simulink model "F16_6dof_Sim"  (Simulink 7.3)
settings: Solver=ode45  StartTime=0.0  StopTime=615.35  RelTol=1e-3
InitFcn:
  | init
StopFcn:
  | pl
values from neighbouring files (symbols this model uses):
  d2r = pi/180    (= 0.0174532925199)    [init.m]    (also in pl.m; LQR_Design.m)
  h0 = 0    [init.m]
  mass = 637    [init.m]
  q = 3    [FCS.m]
  sp = 30    [init.m]
  x0 = 0    [init.m]
  x_cg = -17.29    [init.m]
  x_ref = -17.29    [init.m]
  y_cg = 0    [init.m]
  z_cg = 1.2    [init.m]
undefined symbols (not defined in the file or in its folder): Cl, Cld1, Cld3, Cld4, Cm, Cmd1, Cmd3, Cmd4, Cn, Cnd1, Cnd3, Cnd4, Continuous, CX, CXd1, CXd3, CXd4, CY, CYd1, CYd3, CYd4, CZ, CZd1, CZd3, CZd4, Dryden, F, FCS, ft, km, Light, MIL, r, sigbuilder_block, Thrust
libraries: aerolibasang x3, aerolibwind2 x3, aerolib6dof2 x1, aerolibconvert2 x1, aerolibatmos2 x1, aerolibgravity2 x1, aerolibadyn x1

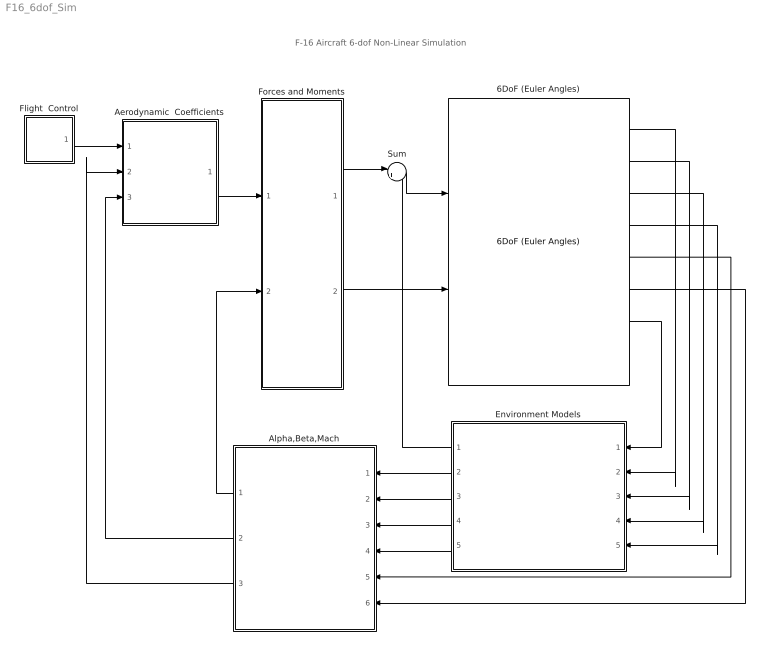
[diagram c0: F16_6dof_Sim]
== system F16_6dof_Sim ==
  note: F-16 Aircraft 6-dof Non-Linear Simulation
  6DoF (Euler Angles) : aerolib6dof2/6DoF (Euler Angles)  SystemSampleTime=-1  units=English (Velocity in ft/s)  mtype=Fixed  rep=Euler Angles  xme_0=[-x0, 0, -h0]  Vm_0=Uvw_0  eul_0=Euler_0  pm_0=pqr_0  mass_0=mass  mass_e=0.5  mass_f=2.0  inertia=inertia  inertia_e=eye(3)  inertia_f=2*eye(3)  k_quat=1.0
  Aerodynamic  Coefficients : Subsystem
  Alpha,Beta,Mach : Subsystem
  Environment Models : Subsystem
  Flight  Control : Subsystem
  Forces and Moments : Subsystem
  Sum : Sum  Inputs=|++  OutDataType=sfix(16)  OutScaling=2^0
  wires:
  6DoF (Euler Angles)/5 -> Alpha,Beta,Mach/5(Vb)
  6DoF (Euler Angles)/1 -> Environment Models/2(Ve)
  6DoF (Euler Angles)/2 -> Environment Models/3(Xe)
  6DoF (Euler Angles)/3 -> Environment Models/4(Euler)
  6DoF (Euler Angles)/4 -> Environment Models/5(DCM)
  Sum/1 -> 6DoF (Euler Angles)/1
  Forces and Moments/1(X,Y,Z) -> Sum/1
  Environment Models/2(Speed of Sound) -> Alpha,Beta,Mach/1(Speed of Sound)
  Environment Models/3(Wind Velocity) -> Alpha,Beta,Mach/2(Wind Velocity)
  Environment Models/4(Air Density) -> Alpha,Beta,Mach/3(Air Density)
  Environment Models/5(Wind Angular Rates) -> Alpha,Beta,Mach/4(Wind Angular Rates)
  Environment Models/1(Fg) -> Sum/2
  Alpha,Beta,Mach/1(qbar) -> Forces and Moments/2(qbar)
  Alpha,Beta,Mach/3(Incid) -> Aerodynamic  Coefficients/2(Incid)
  Alpha,Beta,Mach/2(Mach) -> Aerodynamic  Coefficients/3(Mach)
  6DoF (Euler Angles)/6 -> Alpha,Beta,Mach/6(p,q,r)
  Aerodynamic  Coefficients/1(Coeff) -> Forces and Moments/1(Coeff)
  Forces and Moments/2(LMN) -> 6DoF (Euler Angles)/2
  Flight  Control/1(Deltas) -> Aerodynamic  Coefficients/1(deltas)
  6DoF (Euler Angles)/7 -> Environment Models/1(omgd)

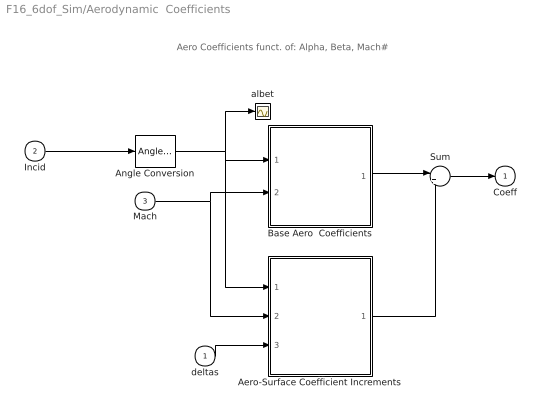
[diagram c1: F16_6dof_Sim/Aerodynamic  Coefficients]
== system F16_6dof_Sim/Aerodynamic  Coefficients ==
  note: Aero Coefficients funct. of: Alpha, Beta, Mach#
  deltas : Inport  OutDataType=sfix(16)  OutScaling=2^0
  Incid : Inport  Port=2  OutDataType=sfix(16)  OutScaling=2^0
  Mach : Inport  Port=3  OutDataType=sfix(16)  OutScaling=2^0
  Aero-Surface Coefficient Increments : Subsystem
  Angle Conversion : aerolibconvert2/Angle Conversion  SystemSampleTime=-1  IU=rad  OU=deg
  Base Aero  Coefficients : Subsystem
  Sum : Sum  Inputs=|++  OutDataType=fixdt(1, 16)  OutScaling=2^0
  albet : Scope
  Coeff : Outport  OutDataType=sfix(16)  OutScaling=2^0  InitialOutput=0
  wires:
  Incid/1 -> Angle Conversion/1
  Angle Conversion/1 -> albet/1, Base Aero  Coefficients/1(albet), Aero-Surface Coefficient Increments/1(albet)
  Mach/1 -> Base Aero  Coefficients/2(Mach), Aero-Surface Coefficient Increments/2(Mach)
  Sum/1 -> Coeff/1
  Base Aero  Coefficients/1(Coeff) -> Sum/1
  Aero-Surface Coefficient Increments/1(Coeff) -> Sum/2
  deltas/1 -> Aero-Surface Coefficient Increments/3(delta)

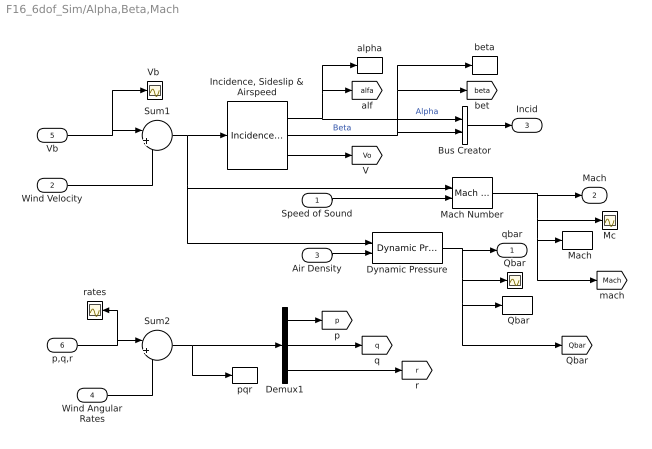
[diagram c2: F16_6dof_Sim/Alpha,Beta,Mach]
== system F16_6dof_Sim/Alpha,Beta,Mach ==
  Speed of Sound : Inport  OutDataType=sfix(16)  OutScaling=2^0
  Wind Velocity : Inport  Port=2  PortDimensions=3  OutDataType=sfix(16)  OutScaling=2^0
  Air Density : Inport  Port=3  OutDataType=sfix(16)  OutScaling=2^0
  Wind Angular Rates : Inport  Port=4  PortDimensions=3  OutDataType=sfix(16)  OutScaling=2^0
  Vb : Inport  Port=5  PortDimensions=3  OutDataType=sfix(16)  OutScaling=2^0
  p,q,r : Inport  Port=6  PortDimensions=3  OutDataType=sfix(16)  OutScaling=2^0
  "  Mach" : ToWorkspace  VariableName=Mach  SampleTime=-1  SaveFormat=Array
  " Qbar" : ToWorkspace  VariableName=Qbar  SampleTime=-1  SaveFormat=Array
  Bus Creator : BusCreator  Inputs=2
  Demux1 : Demux  Outputs=3
  Dynamic Pressure : aerolibasang/Dynamic Pressure  SystemSampleTime=-1
  "Incidence, Sideslip & Airspeed" : aerolibasang/Incidence, Sideslip, & Airspeed  SystemSampleTime=-1
  Mach Number : aerolibasang/Mach Number  SystemSampleTime=-1
  Mc : Scope
  Qbar : Scope
  Sum1 : Sum  Inputs=|+-  OutDataType=sfix(16)  OutScaling=2^0
  Sum2 : Sum  Inputs=|++  OutDataType=sfix(16)  OutScaling=2^0
  "Vb " : Scope
  alpha : ToWorkspace  VariableName=alfa  SampleTime=-1  SaveFormat=Array
  beta : ToWorkspace  VariableName=beta  SampleTime=-1  SaveFormat=Array
  pqr : ToWorkspace  VariableName=pqr  SampleTime=-1  SaveFormat=Array
  rates : Scope
  qbar : Outport  OutDataType=sfix(16)  OutScaling=2^0  InitialOutput=0
  Mach : Outport  Port=2  OutDataType=sfix(16)  OutScaling=2^0
  Incid : Outport  Port=3  OutDataType=sfix(16)  OutScaling=2^0
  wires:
  "Incidence, Sideslip & Airspeed"/3 -> [Vo]
  Dynamic Pressure/1 -> qbar/1, Qbar/1, " Qbar"/1, [Qbar]
  Air Density/1 -> Dynamic Pressure/2
  Mach Number/1 -> Mach/1, Mc/1, "  Mach"/1, [Mach]
  Sum1/1 -> Dynamic Pressure/1, Mach Number/1, "Incidence, Sideslip & Airspeed"/1
  Vb/1 -> Sum1/1, "Vb "/1
  Speed of Sound/1 -> Mach Number/2
  Wind Velocity/1 -> Sum1/2
  "Incidence, Sideslip & Airspeed"/2 -> Bus Creator/2, [beta], beta/1  "Beta"
  Bus Creator/1 -> Incid/1
  "Incidence, Sideslip & Airspeed"/1 -> Bus Creator/1, [alfa], alpha/1  "Alpha"
  p,q,r/1 -> Sum2/1, rates/1
  Wind Angular Rates/1 -> Sum2/2
  Sum2/1 -> Demux1/1, pqr/1
  Demux1/2 -> [q]
  Demux1/3 -> [r]
  Demux1/1 -> [p]

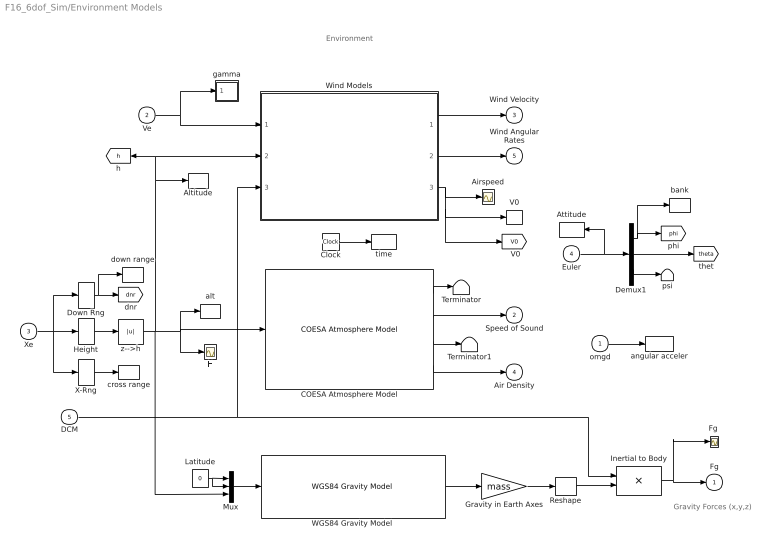
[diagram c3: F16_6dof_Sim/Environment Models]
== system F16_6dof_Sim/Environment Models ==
  note: Gravity Forces (x,y,z)
  note: Environment
  omgd : Inport  OutDataType=sfix(16)  OutScaling=2^0
  Ve : Inport  Port=2  OutDataType=sfix(16)  OutScaling=2^0
  Xe : Inport  Port=3  PortDimensions=3  OutDataType=sfix(16)  OutScaling=2^0
  Euler : Inport  Port=4  OutDataType=sfix(16)  OutScaling=2^0
  DCM : Inport  Port=5  OutDataType=sfix(16)  OutScaling=2^0
  Airspeed : Scope
  Altitude : ToWorkspace  VariableName=Alt  SampleTime=-1  SaveFormat=Array
  Attitude : ToWorkspace  VariableName=Euler  SampleTime=-1  SaveFormat=Array
  COESA Atmosphere Model : aerolibatmos2/COESA Atmosphere Model  SystemSampleTime=-1  units=English (Velocity in ft/s)  spec=1976 COESA-extended U.S. Standard Atmosphere  model=Profile  profile_var=High temperature  profile_percent=1%  profile_alt=5 km (16404 ft)  envelope_var=High temperature  envelope_percent=1%  action=Warning
  Clock : Clock
  Demux1 : Demux  Outputs=3
  Down Rng : Selector  InputPortWidth=3  IndexOptions=Index vector (dialog)  Indices=[1]  OutputSizes=1
  "Fg " : Scope
  Gravity in Earth Axes : Gain  Gain=mass  ParameterDataType=sfix(16)  ParameterScaling=2^0  OutDataType=sfix(16)  OutScaling=2^0
  H : Scope
  Height : Selector  InputPortWidth=3  IndexOptions=Index vector (dialog)  Indices=[3]  OutputSizes=1
  Inertial to Body : Product  Multiplication=Matrix(*)  OutDataType=sfix(16)  OutScaling=2^0
  Latitude : Constant  Value=0  OutDataType=sfix(16)  OutScaling=2^0
  Mux : Mux  Inputs=3
  Reshape : Reshape
  Terminator : Terminator
  Terminator1 : Terminator
  V0 : ToWorkspace  VariableName=V0  SampleTime=-1  SaveFormat=Array
  "WGS84 Gravity Model " : aerolibgravity2/WGS84 Gravity Model   SystemSampleTime=-1  model=WGS84 Taylor Series  units=English  no_atmos=on  precessing=on  jd_loc=off  month=October  day=10  year=2004  no_centrifugal=on  action=None
  Wind Models : Subsystem
  X-Rng : Selector  InputPortWidth=3  IndexOptions=Index vector (dialog)  Indices=[2]  OutputSizes=1
  alt : ToWorkspace  VariableName=alt  SampleTime=-1  SaveFormat=Array
  angular acceler : ToWorkspace  VariableName=omgd  SampleTime=-1  SaveFormat=Array
  bank : ToWorkspace  VariableName=phi  SampleTime=-1  SaveFormat=Array
  cross range : ToWorkspace  VariableName=xrng  SampleTime=-1  SaveFormat=Array
  down range : ToWorkspace  VariableName=dnr  SampleTime=-1  SaveFormat=Array
  gamma : Subsystem
  psi : Terminator
  time : ToWorkspace  VariableName=time  SampleTime=-1  SaveFormat=Array
  z-->h : Abs
  Fg : Outport  OutDataType=sfix(16)  OutScaling=2^0  InitialOutput=0
  Speed of Sound : Outport  Port=2  OutDataType=sfix(16)  OutScaling=2^0  InitialOutput=0
  Wind Velocity : Outport  Port=3  OutDataType=sfix(16)  OutScaling=2^0  InitialOutput=0
  Air Density : Outport  Port=4  OutDataType=sfix(16)  OutScaling=2^0  InitialOutput=0
  Wind Angular Rates : Outport  Port=5  OutDataType=sfix(16)  OutScaling=2^0  InitialOutput=0
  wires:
  Reshape/1 -> Inertial to Body/2
  "WGS84 Gravity Model "/1 -> Gravity in Earth Axes/1
  Gravity in Earth Axes/1 -> Reshape/1
  COESA Atmosphere Model/1 -> Terminator/1
  COESA Atmosphere Model/2 -> Speed of Sound/1
  COESA Atmosphere Model/3 -> Terminator1/1
  COESA Atmosphere Model/4 -> Air Density/1
  DCM/1 -> Inertial to Body/1, Wind Models/3(DCM)
  Inertial to Body/1 -> Fg/1, "Fg "/1
  Mux/1 -> "WGS84 Gravity Model "/1
  Latitude/1 -> Mux/2, Mux/1
  Height/1 -> z-->h/1
  Xe/1 -> Height/1, Down Rng/1, X-Rng/1
  z-->h/1 -> COESA Atmosphere Model/1, H/1, alt/1, Mux/3, Wind Models/2(Altitude), [h], Altitude/1
  Wind Models/2(pg,qg,rg) -> Wind Angular Rates/1
  Wind Models/3(Airspeed) -> Airspeed/1, V0/1, [V0]
  Ve/1 -> Wind Models/1(Ve), gamma/1(Ve)
  Wind Models/1(ug,vg,wg) -> Wind Velocity/1
  Down Rng/1 -> [dnr], down range/1
  Clock/1 -> time/1
  X-Rng/1 -> cross range/1
  omgd/1 -> angular acceler/1
  Euler/1 -> Demux1/1, Attitude/1
  Demux1/2 -> [theta]
  Demux1/1 -> [phi], bank/1
  Demux1/3 -> psi/1

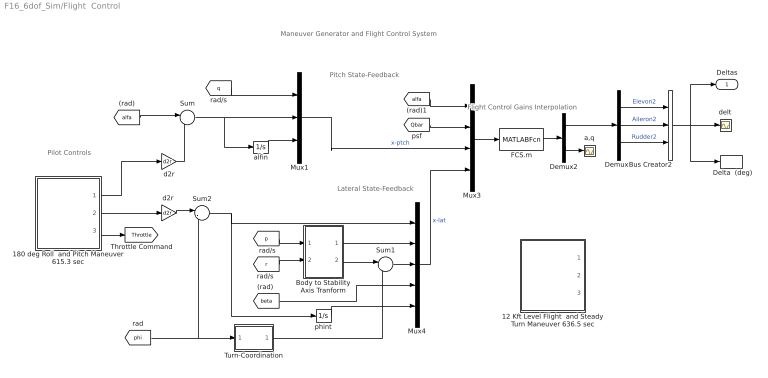
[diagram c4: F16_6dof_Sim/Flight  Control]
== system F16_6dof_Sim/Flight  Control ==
  note: Maneuver Generator and Flight Control System
  note: Flight Control Gains Interpolation
  note: Pilot Controls
  note: Pitch State-Feedback
  note: Lateral State-Feedback
  "  Delta  (deg)" : ToWorkspace  VariableName=delta  SampleTime=-1  SaveFormat=Array
  12 Kft Level Flight  and Steady Turn Maneuver 636.5 sec : Subsystem  Tag=STV Subsys  LoadFcn=sigbuilder_block('load');  StartFcn=sigbuilder_block('start');  StopFcn=sigbuilder_block('stop');  ClipboardFcn=sigbuilder_block('clipboard');
  180 deg Roll  and Pitch Maneuver 615.3 sec : Subsystem  Tag=STV Subsys  LoadFcn=sigbuilder_block('load');  StartFcn=sigbuilder_block('start');  StopFcn=sigbuilder_block('stop');  ClipboardFcn=sigbuilder_block('clipboard');
  Body to Stability Axis Tranform : Subsystem
  Bus Creator2 : BusCreator  Inputs=3
  Demux1 : Demux  Outputs=3
  Demux2 : Demux  Outputs=[3,2]
  FCS.m : MATLABFcn  MATLABFcn=FCS( u(1), u(2), u(3:5), u(6:10) )  OutputDimensions=5
  Mux1 : Mux  Inputs=3
  Mux3 : Mux  Inputs=[1,1, 3, 5]
  Mux4 : Mux  Inputs=5
  Sum : Sum  Inputs=|+-  OutDataType=fixdt(1, 16)  OutScaling=2^0
  Sum1 : Sum  Inputs=|++  OutDataType=fixdt(1, 16)  OutScaling=2^0
  Sum2 : Sum  Inputs=|-+  OutDataType=fixdt(1, 16)  OutScaling=2^0
  Turn-Coordination : Subsystem
  a,q : Scope
  alfin : Integrator
  d2r : Gain  Gain=d2r  ParameterDataType=fixdt(1, 16)  ParameterScaling=2^0  OutDataType=fixdt(1, 16)  OutScaling=2^0
  "d2r " : Gain  Gain=d2r  ParameterDataType=fixdt(1, 16)  ParameterScaling=2^0  OutDataType=fixdt(1, 16)  OutScaling=2^0
  delt : Scope
  phint : Integrator
  Deltas : Outport
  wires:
  Mux1/1 -> Mux3/3  "x-ptch"
  [q] -> Mux1/1
  alfin/1 -> Mux1/3
  Sum/1 -> Mux1/2, alfin/1
  [alfa] -> Sum/1
  d2r/1 -> Sum/2
  Sum2/1 -> phint/1, Mux4/1
  [beta] -> Mux4/4
  phint/1 -> Mux4/5
  180 deg Roll  and Pitch Maneuver 615.3 sec/2(Phi_cmd) -> "d2r "/1
  180 deg Roll  and Pitch Maneuver 615.3 sec/1(Alpha_cmd) -> d2r/1
  180 deg Roll  and Pitch Maneuver 615.3 sec/3(Throttle) -> [Throttle]
  Demux1/1 -> Bus Creator2/1  "Elevon2"
  Bus Creator2/1 -> delt/1, Deltas/1, "  Delta  (deg)"/1
  Demux1/2 -> Bus Creator2/2  "Aileron2"
  Demux1/3 -> Bus Creator2/3  "Rudder2"
  FCS.m/1 -> Demux2/1
  Demux2/1 -> Demux1/1
  Demux2/2 -> a,q/1
  [alfa] -> Mux3/1
  [Qbar] -> Mux3/2
  "d2r "/1 -> Sum2/1
  [phi] -> Sum2/2, Turn-Coordination/1(phi)
  Sum1/1 -> Mux4/3
  Turn-Coordination/1(Rff) -> Sum1/2
  Body to Stability Axis Tranform/2(r_s) -> Sum1/1
  Body to Stability Axis Tranform/1(p_s) -> Mux4/2
  [p] -> Body to Stability Axis Tranform/1(p_b)
  [r] -> Body to Stability Axis Tranform/2(r_b)
  Mux4/1 -> Mux3/4  "x-lat"
  Mux3/1 -> FCS.m/1

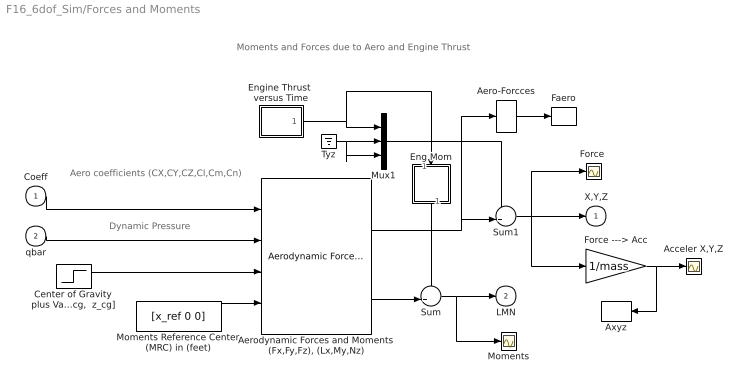
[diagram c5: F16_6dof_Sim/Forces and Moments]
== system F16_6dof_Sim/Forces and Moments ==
  note: Aero coefficients (CX,CY,CZ,Cl,Cm,Cn)
  note: Dynamic Pressure
  note: Moments and Forces due to Aero and Engine Thrust
  Coeff : Inport  OutDataType=sfix(16)  OutScaling=2^0
  qbar : Inport  Port=2  OutDataType=sfix(16)  OutScaling=2^0
  Acceler X,Y,Z : Scope
  Aero-Forcces : Selector  InputPortWidth=3  IndexOptions=Index vector (dialog)  Indices=[3,1,2]  OutputSizes=1
  "Aerodynamic Forces and Moments (Fx,Fy,Fz), (Lx,My,Nz)" : aerolibadyn/Aerodynamic Forces and Moments   SystemSampleTime=-1  inputAxes=Body  outputForceAxes=Body  outputMomentAxes=Body  S=Sref  b=sp  cbar=ch
  Axyz : ToWorkspace  VariableName=Axyz  SampleTime=-1  SaveFormat=Array
  "Center of Gravity plus Variation [x_cg, y_cg,  z_cg]" : Step  Time=100*[1 1 1]  Before="[x_cg, y_cg,  z_cg]"  After="[x_cg,   y_cg+0.0,   z_cg]"
  Eng Mom : Subsystem
  Engine Thrust  versus Time : Subsystem
  Faero : ToWorkspace  VariableName=Flds  SampleTime=-1  SaveFormat=Array
  "Force " : Scope
  Force ---> Acc : Gain  Gain=1/mass  ParameterDataType=sfix(16)  ParameterScaling=2^0  OutDataType=sfix(16)  OutScaling=2^0
  Moments : Scope
  Moments Reference Center (MRC) in (feet) : Constant  Value=[x_ref 0 0]  OutDataType=sfix(16)  OutScaling=2^0
  Mux1 : Mux  Inputs=3
  Sum : Sum  Inputs=++|  OutDataType=fixdt(1, 16)  OutScaling=2^0
  Sum1 : Sum  Inputs=++|  OutDataType=sfix(16)  OutScaling=2^0
  Tyz : Ground
  X,Y,Z : Outport  OutDataType=sfix(16)  OutScaling=2^0  InitialOutput=0
  LMN : Outport  Port=2  OutDataType=sfix(16)  OutScaling=2^0  InitialOutput=0
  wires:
  Coeff/1 -> "Aerodynamic Forces and Moments (Fx,Fy,Fz), (Lx,My,Nz)"/1
  qbar/1 -> "Aerodynamic Forces and Moments (Fx,Fy,Fz), (Lx,My,Nz)"/2
  Sum1/1 -> Force ---> Acc/1, X,Y,Z/1, "Force "/1
  Moments Reference Center (MRC) in (feet)/1 -> "Aerodynamic Forces and Moments (Fx,Fy,Fz), (Lx,My,Nz)"/4
  "Center of Gravity plus Variation [x_cg, y_cg,  z_cg]"/1 -> "Aerodynamic Forces and Moments (Fx,Fy,Fz), (Lx,My,Nz)"/3
  Force ---> Acc/1 -> Acceler X,Y,Z/1, Axyz/1
  Mux1/1 -> Sum1/1
  Tyz/1 -> Mux1/2, Mux1/3
  Engine Thrust  versus Time/1(Thrust) -> Mux1/1, Eng Mom/1(Te)
  Aero-Forcces/1 -> Faero/1
  "Aerodynamic Forces and Moments (Fx,Fy,Fz), (Lx,My,Nz)"/2 -> Sum/2
  "Aerodynamic Forces and Moments (Fx,Fy,Fz), (Lx,My,Nz)"/1 -> Sum1/2, Aero-Forcces/1
  Eng Mom/1(Me) -> Sum/1
  Sum/1 -> LMN/1, Moments/1

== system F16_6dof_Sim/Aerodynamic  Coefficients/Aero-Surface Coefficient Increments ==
  note: Surface Coefficients
  albet : Inport
  Mach : Inport  Port=2
  delta : Inport  Port=3
  Aileron : Subsystem
  Elevon : Subsystem
  Rudder : Subsystem
  Sum : Sum  Inputs=+++  OutDataType=fixdt(1, 16)  OutScaling=2^0
  Coeff : Outport
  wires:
  Elevon/1(Coeff) -> Sum/1
  delta/1 -> Elevon/3(delta), Aileron/3(delta), Rudder/3(delta)
  albet/1 -> Elevon/1(albet), Aileron/1(albet), Rudder/1(albet)
  Mach/1 -> Elevon/2(Mach), Aileron/2(Mach), Rudder/2(Mach)
  Sum/1 -> Coeff/1
  Aileron/1(Coeff) -> Sum/2
  Rudder/1(Coeff) -> Sum/3

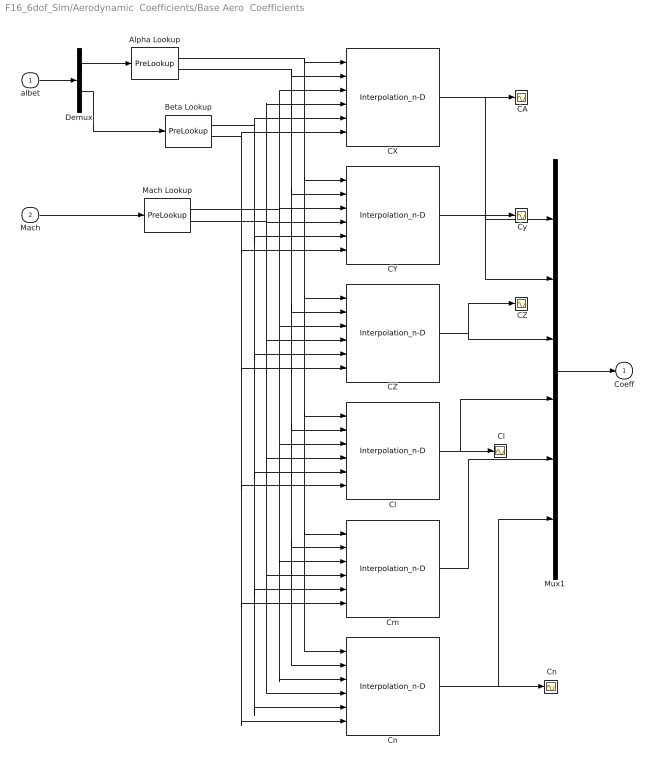
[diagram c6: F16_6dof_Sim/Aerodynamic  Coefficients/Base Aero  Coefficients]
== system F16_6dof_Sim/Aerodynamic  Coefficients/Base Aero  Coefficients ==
  albet : Inport  OutDataType=sfix(16)  OutScaling=2^0
  Mach : Inport  Port=2  OutDataType=sfix(16)  OutScaling=2^0
  " CA" : Scope
  " CZ" : Scope
  " Cl" : Scope
  " Cn" : Scope
  " Cy" : Scope
  Alpha Lookup : PreLookup  BreakpointsData=Alfas  BeginIndexSearchUsingPreviousIndexResult=on  ProcessOutOfRangeInput=Linear extrapolation  IndexDataType=sfix(16)  FractionDataType=sfix(16)  FractionScaling=2^0
  Beta Lookup : PreLookup  BreakpointsData=Betas  BeginIndexSearchUsingPreviousIndexResult=on  ProcessOutOfRangeInput=Linear extrapolation  IndexDataType=sfix(16)  FractionDataType=sfix(16)  FractionScaling=2^0
  CX : Interpolation_n-D  NumberOfTableDimensions=3  Table=CX  CheckIndexInCode=off  OutDataType=sfix(16)  OutScaling=2^0
  CY : Interpolation_n-D  NumberOfTableDimensions=3  Table=CY  CheckIndexInCode=off  OutDataType=sfix(16)  OutScaling=2^0
  CZ : Interpolation_n-D  NumberOfTableDimensions=3  Table=CZ  CheckIndexInCode=off  OutDataType=sfix(16)  OutScaling=2^0
  Cl : Interpolation_n-D  NumberOfTableDimensions=3  Table=Cl  CheckIndexInCode=off  OutDataTypeMode=double  OutDataType=sfix(16)  OutScaling=2^0  OutDataTypeStr=double
  Cm : Interpolation_n-D  NumberOfTableDimensions=3  Table=Cm  CheckIndexInCode=off  OutDataType=sfix(16)  OutScaling=2^0
  Cn : Interpolation_n-D  NumberOfTableDimensions=3  Table=Cn  CheckIndexInCode=off  OutDataType=sfix(16)  OutScaling=2^0
  Demux : Demux  Outputs=2
  Mach Lookup : PreLookup  BreakpointsData=Machs  BeginIndexSearchUsingPreviousIndexResult=on  ProcessOutOfRangeInput=Linear extrapolation  IndexDataType=sfix(16)  FractionDataType=sfix(16)  FractionScaling=2^0
  Mux1 : Mux  Inputs=6
  Coeff : Outport  OutDataType=sfix(16)  OutScaling=2^0  InitialOutput=0
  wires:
  Demux/1 -> Alpha Lookup/1
  CX/1 -> Mux1/1, " CA"/1
  CY/1 -> Mux1/2, " Cy"/1
  CZ/1 -> Mux1/3, " CZ"/1
  Cl/1 -> Mux1/4, " Cl"/1
  Cm/1 -> Mux1/5
  Cn/1 -> Mux1/6, " Cn"/1
  Alpha Lookup/1 -> CX/1, CY/1, Cm/1, Cn/1, Cl/1, CZ/1
  Alpha Lookup/2 -> CX/2, CY/2, CZ/2, Cl/2, Cm/2, Cn/2
  Mach Lookup/1 -> CY/3, Cm/3, Cn/3, Cl/3, CZ/3, CX/3
  Mach Lookup/2 -> CY/4, Cm/4, Cn/4, Cl/4, CZ/4, CX/4
  Beta Lookup/1 -> CX/5, Cm/5, Cn/5, Cl/5, CZ/5, CY/5
  Beta Lookup/2 -> CX/6, CY/6, Cm/6, Cn/6, Cl/6, CZ/6
  Mux1/1 -> Coeff/1
  Demux/2 -> Beta Lookup/1
  albet/1 -> Demux/1
  Mach/1 -> Mach Lookup/1

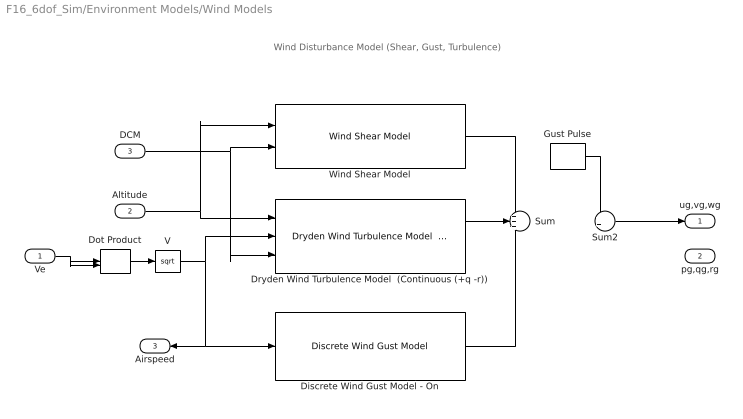
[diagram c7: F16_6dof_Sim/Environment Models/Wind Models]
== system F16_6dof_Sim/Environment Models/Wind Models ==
  note: Wind Disturbance Model (Shear, Gust, Turbulence)
  Ve : Inport  OutDataType=sfix(16)  OutScaling=2^0
  Altitude : Inport  Port=2  OutDataType=sfix(16)  OutScaling=2^0
  DCM : Inport  Port=3  OutDataType=sfix(16)  OutScaling=2^0
  Discrete Wind Gust Model - On : aerolibwind2/Discrete Wind Gust Model  SystemSampleTime=-1  units=English (Velocity in ft/s)  Gx=on  Gy=on  Gz=on  t_0=20  d_m=[120 120 80]  v_m=[3.5 3.0 3.0]
  Dot Product : DotProduct  OutDataType=sfix(16)  OutScaling=2^-10  SaturateOnIntegerOverflow=on
  Dryden Wind Turbulence Model  (Continuous (+q -r)) : aerolibwind2/Dryden Wind Turbulence Model  (Continuous (+q -r))  SystemSampleTime=-1  units=English (Velocity in ft/s)  spec=MIL-F-8785C  model=Continuous Dryden (+q -r)  W20=5  Wdeg=0  TurbProb=10^-2 - Light  L_high=533.4  Wingspan=4  ts=0.1  Seed=[23341 23342 23343 23344]  T_on=on
  Gust Pulse : DiscretePulseGenerator  PulseType=Time based  Amplitude=[0, 0, 0]  Period=[100, 100, 100]  PulseWidth=1  PhaseDelay=0  SampleTime=1
  Sum : Sum  Inputs=+++  OutDataType=sfix(16)  OutScaling=2^0
  Sum2 : Sum  Inputs=++|  OutDataType=sfix(16)  OutScaling=2^0
  V : Math  Operator=sqrt  OutDataType=sfix(16)  OutScaling=2^0
  Wind Shear Model : aerolibwind2/Wind Shear Model  SystemSampleTime=-1  units=English (Velocity in ft/s)  phase=Category C - Terminal Flight Phase  W_20=1  Wdeg=0
  ug,vg,wg : Outport  OutDataType=sfix(16)  OutScaling=2^0
  pg,qg,rg : Outport  Port=2  OutDataType=sfix(16)  OutScaling=2^0
  Airspeed : Outport  Port=3  OutDataType=sfix(16)  OutScaling=2^0
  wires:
  Dryden Wind Turbulence Model  (Continuous (+q -r))/1 -> Sum/2
  Discrete Wind Gust Model - On/1 -> Sum/3
  Wind Shear Model/1 -> Sum/1
  DCM/1 -> Wind Shear Model/2, Dryden Wind Turbulence Model  (Continuous (+q -r))/3
  Altitude/1 -> Dryden Wind Turbulence Model  (Continuous (+q -r))/1, Wind Shear Model/1
  Dot Product/1 -> V/1
  Ve/1 -> Dot Product/1, Dot Product/2
  V/1 -> Dryden Wind Turbulence Model  (Continuous (+q -r))/2, Discrete Wind Gust Model - On/1, Airspeed/1
  Sum2/1 -> ug,vg,wg/1
  Gust Pulse/1 -> Sum2/1
  Sum/1 -> ?
  Dryden Wind Turbulence Model  (Continuous (+q -r))/2 -> ?

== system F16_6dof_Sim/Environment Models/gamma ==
  Ve : Inport
  -1 : Gain  Gain=-1  ParameterDataType=sfix(16)  ParameterScaling=2^0  OutDataType=sfix(16)  OutScaling=2^0
  57.2 : Gain  Gain=180/pi  ParameterDataType=sfix(16)  ParameterScaling=2^0  OutDataType=sfix(16)  OutScaling=2^0
  Vx : Selector  InputPortWidth=3  IndexOptions=Index vector (dialog)  Indices=[1]  OutputSizes=1
  Vz : Selector  InputPortWidth=3  IndexOptions=Index vector (dialog)  Indices=[3]  OutputSizes=1
  atan : Trigonometry  Operator=atan2
  "gam " : Scope
  gama : ToWorkspace  VariableName=gama  SampleTime=-1  SaveFormat=Array
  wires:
  Vz/1 -> atan/1
  Vx/1 -> atan/2
  atan/1 -> 57.2/1
  57.2/1 -> "gam "/1, gama/1
  -1/1 -> Vz/1
  Ve/1 -> -1/1, Vx/1

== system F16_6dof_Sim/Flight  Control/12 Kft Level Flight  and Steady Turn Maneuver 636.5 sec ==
  Demux : Demux  Tag=STV Demux  Outputs=3
  FromWs : FromWorkspace  Tag=STV FromWs  VariableName=tuvar  SampleTime=0  SigBuilderData=DataTag0  VnvData=DataTag1
  Alpha_cmd : Outport  Tag=STV Outport
  Phi_cmd : Outport  Tag=STV Outport  Port=2
  Throttle : Outport  Tag=STV Outport  Port=3
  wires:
  FromWs/1 -> Demux/1
  Demux/1 -> Alpha_cmd/1
  Demux/2 -> Phi_cmd/1
  Demux/3 -> Throttle/1

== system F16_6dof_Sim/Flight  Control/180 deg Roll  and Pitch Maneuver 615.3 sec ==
  Demux : Demux  Tag=STV Demux  Outputs=3
  FromWs : FromWorkspace  Tag=STV FromWs  VariableName=tuvar  SampleTime=0  SigBuilderData=DataTag2  VnvData=DataTag3
  Alpha_cmd : Outport  Tag=STV Outport
  Phi_cmd : Outport  Tag=STV Outport  Port=2
  Throttle : Outport  Tag=STV Outport  Port=3
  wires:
  FromWs/1 -> Demux/1
  Demux/1 -> Alpha_cmd/1
  Demux/2 -> Phi_cmd/1
  Demux/3 -> Throttle/1

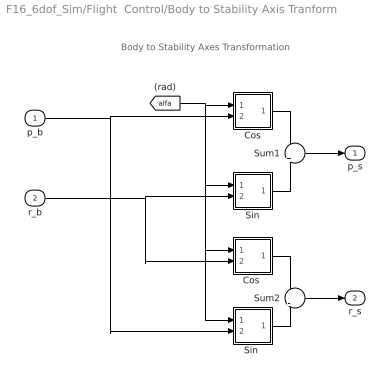
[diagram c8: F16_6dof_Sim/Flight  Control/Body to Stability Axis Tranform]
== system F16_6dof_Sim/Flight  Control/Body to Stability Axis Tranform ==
  note: Body to Stability Axes Transformation
  p_b : Inport  OutDataType=sfix(16)  OutScaling=2^0
  r_b : Inport  Port=2  OutDataType=sfix(16)  OutScaling=2^0
  Cos : Subsystem
  "Cos " : Subsystem
  Sin : Subsystem
  "Sin " : Subsystem
  Sum1 : Sum  Inputs=+|+  OutDataType=sfix(16)  OutScaling=2^0
  Sum2 : Sum  Inputs=+|-  OutDataType=sfix(16)  OutScaling=2^0
  p_s : Outport  OutDataType=sfix(16)  OutScaling=2^0
  r_s : Outport  Port=2  OutDataType=sfix(16)  OutScaling=2^0
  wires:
  Sum1/1 -> p_s/1
  Sum2/1 -> r_s/1
  p_b/1 -> Cos/2(in), "Sin "/2(in)
  r_b/1 -> Sin/2(in), "Cos "/2(in)
  Sin/1(sa) -> Sum1/2
  "Cos "/1(ca) -> Sum2/1
  "Sin "/1(sa) -> Sum2/2
  Cos/1(ca) -> Sum1/1
  [alfa] -> Cos/1(alf), Sin/1(alf), "Cos "/1(alf), "Sin "/1(alf)

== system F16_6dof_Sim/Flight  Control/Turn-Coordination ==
  note: Turn Coordination Rff = (g/V0)*sin(phi)
  phi : Inport
  Divide : Product  Inputs=**/  OutDataType=fixdt(1, 16)  OutScaling=2^-10
  g : Constant  Value=-32.174  OutDataType=fixdt(1, 16)  OutScaling=2^0
  sin : Trigonometry
  Rff : Outport
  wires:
  [V0] -> Divide/3
  sin/1 -> Divide/1
  phi/1 -> sin/1
  Divide/1 -> Rff/1
  g/1 -> Divide/2

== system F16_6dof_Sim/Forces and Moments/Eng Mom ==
  Te : Inport
  0 : Ground
  Mux2 : Mux  Inputs=3
  ly : Gain  Gain=-y_cg  ParameterDataType=sfix(16)  ParameterScaling=2^0  OutDataType=sfix(16)  OutScaling=2^0
  lz : Gain  Gain=-z_cg  ParameterDataType=sfix(16)  ParameterScaling=2^0  OutDataType=sfix(16)  OutScaling=2^0
  Me : Outport
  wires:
  lz/1 -> Mux2/2
  ly/1 -> Mux2/1
  0/1 -> Mux2/3
  Te/1 -> lz/1, ly/1
  Mux2/1 -> Me/1

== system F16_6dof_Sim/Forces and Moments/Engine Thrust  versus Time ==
  note: Thrust as a Funct. of Throttle Control Altitude, and Mach Number
  Mux1 : Mux  Inputs=3
  T : Scope
  Throttle : ToWorkspace  VariableName=Thro  SampleTime=-1  SaveFormat=Array
  Thrust.m : MATLABFcn  MATLABFcn=Thrust( u(1), u(2), u(3) )  OutputDimensions=1
  thrust : ToWorkspace  VariableName=Teng  SampleTime=-1  SaveFormat=Array
  Thrust : Outport  OutDataType=sfix(16)  OutScaling=2^0  InitialOutput=0
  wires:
  [h] -> Mux1/2
  [Mach] -> Mux1/3
  [Throttle] -> Throttle/1, Mux1/1
  Thrust.m/1 -> thrust/1, Thrust/1, T/1
  Mux1/1 -> Thrust.m/1

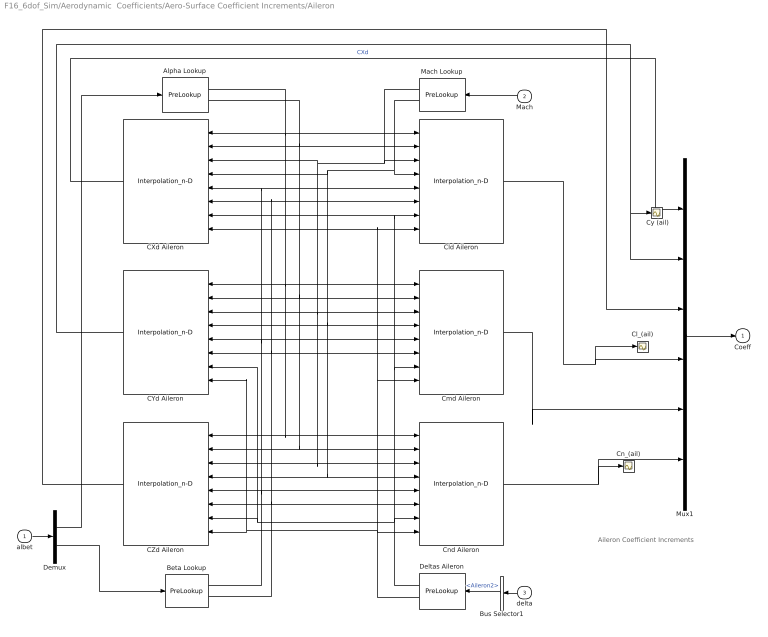
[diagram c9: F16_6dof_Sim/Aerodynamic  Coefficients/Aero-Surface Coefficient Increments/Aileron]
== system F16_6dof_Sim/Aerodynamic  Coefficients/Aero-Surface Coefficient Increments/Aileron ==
  note: Aileron Coefficient Increments
  albet : Inport  OutDataType=sfix(16)  OutScaling=2^0
  Mach : Inport  Port=2  OutDataType=sfix(16)  OutScaling=2^0
  delta : Inport  Port=3  OutDataType=sfix(16)  OutScaling=2^0
  " Cy (ail)" : Scope
  Alpha Lookup : PreLookup  BreakpointsData=Alfas  BeginIndexSearchUsingPreviousIndexResult=on  ProcessOutOfRangeInput=Linear extrapolation  IndexDataType=sfix(16)  FractionDataType=sfix(16)  FractionScaling=2^0
  Beta Lookup : PreLookup  BreakpointsData=Betas  BeginIndexSearchUsingPreviousIndexResult=on  ProcessOutOfRangeInput=Linear extrapolation  IndexDataType=sfix(16)  FractionDataType=sfix(16)  FractionScaling=2^0
  Bus Selector1 : BusSelector  OutputSignals=Aileron2
  CXd Aileron : Interpolation_n-D  NumberOfTableDimensions=4  Table=CXd3  CheckIndexInCode=off  OutDataType=sfix(16)  OutScaling=2^0
  CYd Aileron : Interpolation_n-D  NumberOfTableDimensions=4  Table=CYd3  CheckIndexInCode=off  OutDataType=sfix(16)  OutScaling=2^0
  CZd Aileron : Interpolation_n-D  NumberOfTableDimensions=4  Table=CZd3  CheckIndexInCode=off  OutDataType=sfix(16)  OutScaling=2^0
  Cl_(ail) : Scope
  Cld Aileron : Interpolation_n-D  NumberOfTableDimensions=4  Table=Cld3  CheckIndexInCode=off  OutDataType=sfix(16)  OutScaling=2^0
  Cmd Aileron : Interpolation_n-D  NumberOfTableDimensions=4  Table=Cmd3  CheckIndexInCode=off  OutDataType=sfix(16)  OutScaling=2^0
  Cn_(ail) : Scope
  Cnd Aileron : Interpolation_n-D  NumberOfTableDimensions=4  Table=Cnd3  CheckIndexInCode=off  OutDataType=sfix(16)  OutScaling=2^0
  Deltas Aileron : PreLookup  BreakpointsData=Deltas3  BeginIndexSearchUsingPreviousIndexResult=on  ProcessOutOfRangeInput=Linear extrapolation  IndexDataType=sfix(16)  FractionDataType=sfix(16)  FractionScaling=2^0
  Demux : Demux  Outputs=2
  Mach Lookup : PreLookup  BreakpointsData=Machs  BeginIndexSearchUsingPreviousIndexResult=on  ProcessOutOfRangeInput=Linear extrapolation  IndexDataType=sfix(16)  FractionDataType=sfix(16)  FractionScaling=2^0
  Mux1 : Mux  Inputs=6
  Coeff : Outport  OutDataType=sfix(16)  OutScaling=2^0  InitialOutput=0
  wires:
  CZd Aileron/1 -> Mux1/3
  CYd Aileron/1 -> Mux1/2, " Cy (ail)"/1
  CXd Aileron/1 -> Mux1/1  "CXd"
  delta/1 -> Bus Selector1/1
  Demux/2 -> Beta Lookup/1
  Mach/1 -> Mach Lookup/1
  Demux/1 -> Alpha Lookup/1
  Cld Aileron/1 -> Mux1/4, Cl_(ail)/1
  Cmd Aileron/1 -> Mux1/5
  Cnd Aileron/1 -> Mux1/6, Cn_(ail)/1
  Mux1/1 -> Coeff/1
  Deltas Aileron/2 -> CXd Aileron/8, Cld Aileron/8, Cmd Aileron/8, Cnd Aileron/8, CYd Aileron/8, CZd Aileron/8
  Deltas Aileron/1 -> CXd Aileron/7, Cld Aileron/7, Cmd Aileron/7, Cnd Aileron/7, CYd Aileron/7, CZd Aileron/7
  Beta Lookup/2 -> Cld Aileron/6, CXd Aileron/6, Cmd Aileron/6, CYd Aileron/6, Cnd Aileron/6, CZd Aileron/6
  Beta Lookup/1 -> Cld Aileron/5, CXd Aileron/5, Cmd Aileron/5, CYd Aileron/5, Cnd Aileron/5, CZd Aileron/5
  Mach Lookup/2 -> Cnd Aileron/4, CZd Aileron/4, Cmd Aileron/4, CYd Aileron/4, CXd Aileron/4, Cld Aileron/4
  Mach Lookup/1 -> Cnd Aileron/3, CZd Aileron/3, Cmd Aileron/3, CYd Aileron/3, CXd Aileron/3, Cld Aileron/3
  Alpha Lookup/2 -> Cnd Aileron/2, CZd Aileron/2, Cmd Aileron/2, CYd Aileron/2, Cld Aileron/2, CXd Aileron/2
  Alpha Lookup/1 -> Cnd Aileron/1, CZd Aileron/1, Cmd Aileron/1, CYd Aileron/1, Cld Aileron/1, CXd Aileron/1
  albet/1 -> Demux/1
  Bus Selector1/1 -> Deltas Aileron/1  "<Aileron2>"

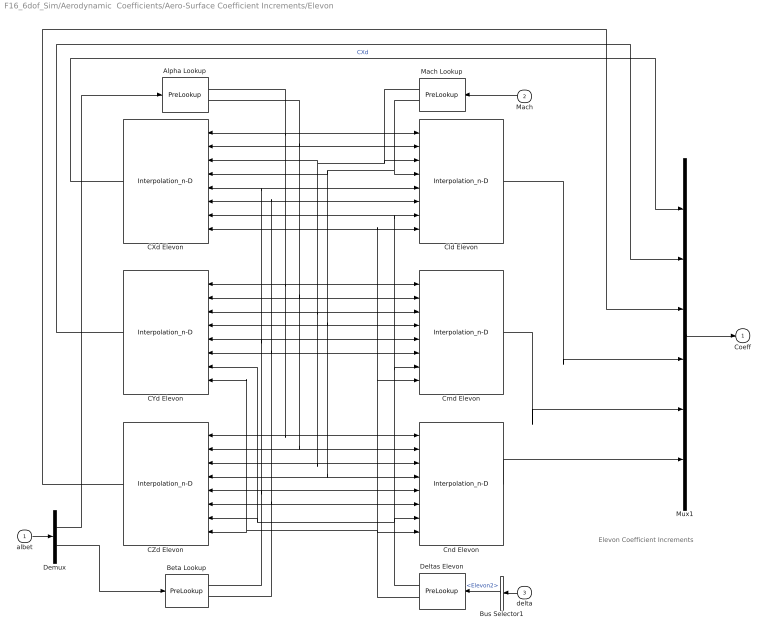
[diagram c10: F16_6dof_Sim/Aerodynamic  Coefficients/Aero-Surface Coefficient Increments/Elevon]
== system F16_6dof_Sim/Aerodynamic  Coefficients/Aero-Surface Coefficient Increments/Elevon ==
  note: Elevon Coefficient Increments
  albet : Inport  OutDataType=sfix(16)  OutScaling=2^0
  Mach : Inport  Port=2  OutDataType=sfix(16)  OutScaling=2^0
  delta : Inport  Port=3  OutDataType=sfix(16)  OutScaling=2^0
  Alpha Lookup : PreLookup  BreakpointsData=Alfas  BeginIndexSearchUsingPreviousIndexResult=on  ProcessOutOfRangeInput=Linear extrapolation  IndexDataType=sfix(16)  FractionDataType=sfix(16)  FractionScaling=2^0
  Beta Lookup : PreLookup  BreakpointsData=Betas  BeginIndexSearchUsingPreviousIndexResult=on  ProcessOutOfRangeInput=Linear extrapolation  IndexDataType=sfix(16)  FractionDataType=sfix(16)  FractionScaling=2^0
  Bus Selector1 : BusSelector  OutputSignals=Elevon2
  CXd Elevon : Interpolation_n-D  NumberOfTableDimensions=4  Table=CXd1  CheckIndexInCode=off  OutDataType=sfix(16)  OutScaling=2^0
  CYd Elevon : Interpolation_n-D  NumberOfTableDimensions=4  Table=CYd1  CheckIndexInCode=off  OutDataType=sfix(16)  OutScaling=2^0
  CZd Elevon : Interpolation_n-D  NumberOfTableDimensions=4  Table=CZd1  CheckIndexInCode=off  OutDataType=sfix(16)  OutScaling=2^0
  Cld Elevon : Interpolation_n-D  NumberOfTableDimensions=4  Table=Cld1  CheckIndexInCode=off  OutDataType=sfix(16)  OutScaling=2^0
  Cmd Elevon : Interpolation_n-D  NumberOfTableDimensions=4  Table=Cmd1  CheckIndexInCode=off  OutDataType=sfix(16)  OutScaling=2^0
  Cnd Elevon : Interpolation_n-D  NumberOfTableDimensions=4  Table=Cnd1  CheckIndexInCode=off  OutDataType=sfix(16)  OutScaling=2^0
  Deltas Elevon : PreLookup  BreakpointsData=Deltas1  BeginIndexSearchUsingPreviousIndexResult=on  ProcessOutOfRangeInput=Linear extrapolation  IndexDataType=sfix(16)  FractionDataType=sfix(16)  FractionScaling=2^0
  Demux : Demux  Outputs=2
  Mach Lookup : PreLookup  BreakpointsData=Machs  BeginIndexSearchUsingPreviousIndexResult=on  ProcessOutOfRangeInput=Linear extrapolation  IndexDataType=sfix(16)  FractionDataType=sfix(16)  FractionScaling=2^0
  Mux1 : Mux  Inputs=6
  Coeff : Outport  OutDataType=sfix(16)  OutScaling=2^0  InitialOutput=0
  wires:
  CZd Elevon/1 -> Mux1/3
  CYd Elevon/1 -> Mux1/2
  CXd Elevon/1 -> Mux1/1  "CXd"
  Demux/2 -> Beta Lookup/1
  Mach/1 -> Mach Lookup/1
  Demux/1 -> Alpha Lookup/1
  Cld Elevon/1 -> Mux1/4
  Cmd Elevon/1 -> Mux1/5
  Cnd Elevon/1 -> Mux1/6
  Mux1/1 -> Coeff/1
  Deltas Elevon/2 -> CXd Elevon/8, Cld Elevon/8, Cmd Elevon/8, Cnd Elevon/8, CYd Elevon/8, CZd Elevon/8
  Deltas Elevon/1 -> CXd Elevon/7, Cld Elevon/7, Cmd Elevon/7, Cnd Elevon/7, CYd Elevon/7, CZd Elevon/7
  Beta Lookup/2 -> Cld Elevon/6, CXd Elevon/6, Cmd Elevon/6, CYd Elevon/6, Cnd Elevon/6, CZd Elevon/6
  Beta Lookup/1 -> Cld Elevon/5, CXd Elevon/5, Cmd Elevon/5, CYd Elevon/5, Cnd Elevon/5, CZd Elevon/5
  Mach Lookup/2 -> Cnd Elevon/4, CZd Elevon/4, Cmd Elevon/4, CYd Elevon/4, CXd Elevon/4, Cld Elevon/4
  Mach Lookup/1 -> Cnd Elevon/3, CZd Elevon/3, Cmd Elevon/3, CYd Elevon/3, CXd Elevon/3, Cld Elevon/3
  Alpha Lookup/2 -> Cnd Elevon/2, CZd Elevon/2, Cmd Elevon/2, CYd Elevon/2, Cld Elevon/2, CXd Elevon/2
  Alpha Lookup/1 -> Cnd Elevon/1, CZd Elevon/1, Cmd Elevon/1, CYd Elevon/1, Cld Elevon/1, CXd Elevon/1
  albet/1 -> Demux/1
  Bus Selector1/1 -> Deltas Elevon/1  "<Elevon2>"
  delta/1 -> Bus Selector1/1

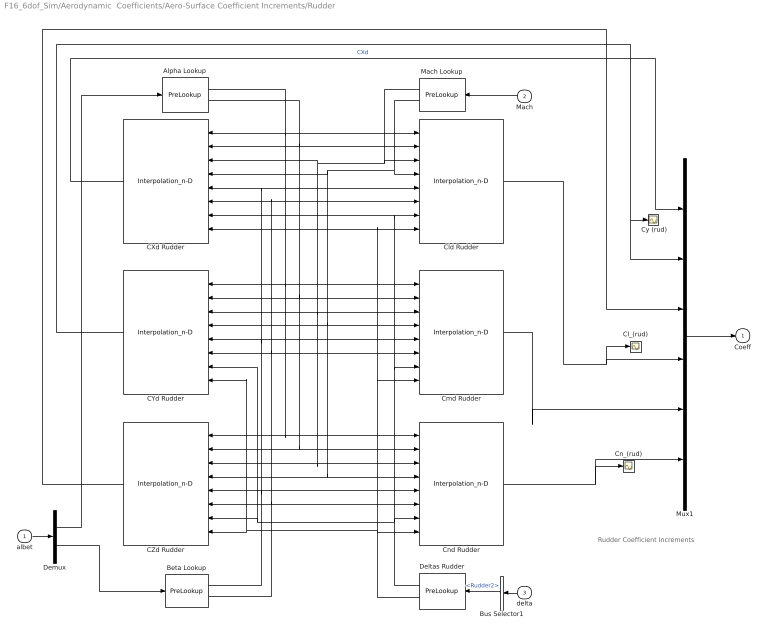
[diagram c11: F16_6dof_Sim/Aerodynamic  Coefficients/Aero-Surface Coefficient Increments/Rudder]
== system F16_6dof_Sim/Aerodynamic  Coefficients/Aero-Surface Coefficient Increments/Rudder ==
  note: Rudder Coefficient Increments
  albet : Inport  OutDataType=sfix(16)  OutScaling=2^0
  Mach : Inport  Port=2  OutDataType=sfix(16)  OutScaling=2^0
  delta : Inport  Port=3  OutDataType=sfix(16)  OutScaling=2^0
  " Cy (rud)" : Scope
  Alpha Lookup : PreLookup  BreakpointsData=Alfas  BeginIndexSearchUsingPreviousIndexResult=on  ProcessOutOfRangeInput=Linear extrapolation  IndexDataType=sfix(16)  FractionDataType=sfix(16)  FractionScaling=2^0
  Beta Lookup : PreLookup  BreakpointsData=Betas  BeginIndexSearchUsingPreviousIndexResult=on  ProcessOutOfRangeInput=Linear extrapolation  IndexDataType=sfix(16)  FractionDataType=sfix(16)  FractionScaling=2^0
  Bus Selector1 : BusSelector  OutputSignals=Rudder2
  CXd Rudder : Interpolation_n-D  NumberOfTableDimensions=4  Table=CXd4  CheckIndexInCode=off  OutDataType=sfix(16)  OutScaling=2^0
  CYd Rudder : Interpolation_n-D  NumberOfTableDimensions=4  Table=CYd4  CheckIndexInCode=off  OutDataType=sfix(16)  OutScaling=2^0
  CZd Rudder : Interpolation_n-D  NumberOfTableDimensions=4  Table=CZd4  CheckIndexInCode=off  OutDataType=sfix(16)  OutScaling=2^0
  Cl_(rud) : Scope
  Cld Rudder : Interpolation_n-D  NumberOfTableDimensions=4  Table=Cld4  CheckIndexInCode=off  OutDataType=sfix(16)  OutScaling=2^0
  Cmd Rudder : Interpolation_n-D  NumberOfTableDimensions=4  Table=Cmd4  CheckIndexInCode=off  OutDataType=sfix(16)  OutScaling=2^0
  Cn_(rud) : Scope
  Cnd Rudder : Interpolation_n-D  NumberOfTableDimensions=4  Table=Cnd4  CheckIndexInCode=off  OutDataType=sfix(16)  OutScaling=2^0
  Deltas Rudder : PreLookup  BreakpointsData=Deltas4  BeginIndexSearchUsingPreviousIndexResult=on  ProcessOutOfRangeInput=Linear extrapolation  IndexDataType=sfix(16)  FractionDataType=sfix(16)  FractionScaling=2^0
  Demux : Demux  Outputs=2
  Mach Lookup : PreLookup  BreakpointsData=Machs  BeginIndexSearchUsingPreviousIndexResult=on  ProcessOutOfRangeInput=Linear extrapolation  IndexDataType=sfix(16)  FractionDataType=sfix(16)  FractionScaling=2^0
  Mux1 : Mux  Inputs=6
  Coeff : Outport  OutDataType=sfix(16)  OutScaling=2^0  InitialOutput=0
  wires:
  CZd Rudder/1 -> Mux1/3
  CYd Rudder/1 -> Mux1/2, " Cy (rud)"/1
  CXd Rudder/1 -> Mux1/1  "CXd"
  delta/1 -> Bus Selector1/1
  Demux/2 -> Beta Lookup/1
  Mach/1 -> Mach Lookup/1
  Demux/1 -> Alpha Lookup/1
  Cld Rudder/1 -> Mux1/4, Cl_(rud)/1
  Cmd Rudder/1 -> Mux1/5
  Cnd Rudder/1 -> Mux1/6, Cn_(rud)/1
  Mux1/1 -> Coeff/1
  Deltas Rudder/2 -> CXd Rudder/8, Cld Rudder/8, Cmd Rudder/8, Cnd Rudder/8, CYd Rudder/8, CZd Rudder/8
  Deltas Rudder/1 -> CXd Rudder/7, Cld Rudder/7, Cmd Rudder/7, Cnd Rudder/7, CYd Rudder/7, CZd Rudder/7
  Beta Lookup/2 -> Cld Rudder/6, CXd Rudder/6, Cmd Rudder/6, CYd Rudder/6, Cnd Rudder/6, CZd Rudder/6
  Beta Lookup/1 -> Cld Rudder/5, CXd Rudder/5, Cmd Rudder/5, CYd Rudder/5, Cnd Rudder/5, CZd Rudder/5
  Mach Lookup/2 -> Cnd Rudder/4, CZd Rudder/4, Cmd Rudder/4, CYd Rudder/4, CXd Rudder/4, Cld Rudder/4
  Mach Lookup/1 -> Cnd Rudder/3, CZd Rudder/3, Cmd Rudder/3, CYd Rudder/3, CXd Rudder/3, Cld Rudder/3
  Alpha Lookup/2 -> Cnd Rudder/2, CZd Rudder/2, Cmd Rudder/2, CYd Rudder/2, Cld Rudder/2, CXd Rudder/2
  Alpha Lookup/1 -> Cnd Rudder/1, CZd Rudder/1, Cmd Rudder/1, CYd Rudder/1, Cld Rudder/1, CXd Rudder/1
  albet/1 -> Demux/1
  Bus Selector1/1 -> Deltas Rudder/1  "<Rudder2>"

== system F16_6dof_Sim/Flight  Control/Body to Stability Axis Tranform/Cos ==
  alf : Inport
  in : Inport  Port=2  OutDataType=sfix(16)  OutScaling=2^0
  Product : Product  OutDataType=fixdt(1, 16)  OutScaling=2^0
  cos : Trigonometry  Operator=cos
  ca : Outport
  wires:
  cos/1 -> Product/1
  in/1 -> Product/2
  alf/1 -> cos/1
  Product/1 -> ca/1

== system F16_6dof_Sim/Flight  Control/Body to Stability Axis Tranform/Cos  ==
  alf : Inport
  in : Inport  Port=2  OutDataType=sfix(16)  OutScaling=2^0
  Product : Product  OutDataType=fixdt(1, 16)  OutScaling=2^0
  cos : Trigonometry  Operator=cos
  ca : Outport
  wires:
  cos/1 -> Product/1
  in/1 -> Product/2
  alf/1 -> cos/1
  Product/1 -> ca/1

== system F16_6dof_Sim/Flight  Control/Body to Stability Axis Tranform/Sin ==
  alf : Inport
  in : Inport  Port=2  OutDataType=sfix(16)  OutScaling=2^0
  Product : Product  OutDataType=fixdt(1, 16)  OutScaling=2^0
  sin : Trigonometry
  sa : Outport
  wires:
  sin/1 -> Product/1
  in/1 -> Product/2
  alf/1 -> sin/1
  Product/1 -> sa/1

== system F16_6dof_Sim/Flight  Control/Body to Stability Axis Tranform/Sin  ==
  alf : Inport
  in : Inport  Port=2  OutDataType=sfix(16)  OutScaling=2^0
  Product : Product  OutDataType=fixdt(1, 16)  OutScaling=2^0
  sin : Trigonometry
  sa : Outport
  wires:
  sin/1 -> Product/1
  in/1 -> Product/2
  alf/1 -> sin/1
  Product/1 -> sa/1
